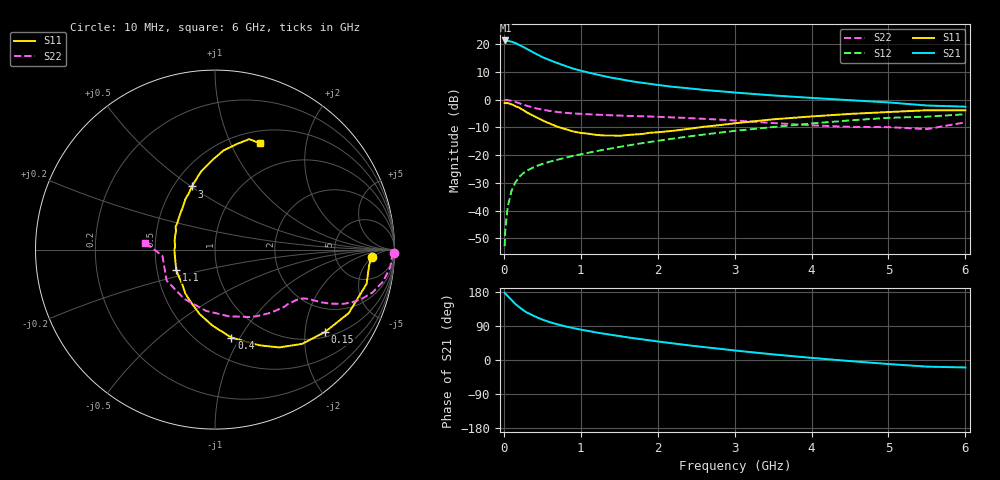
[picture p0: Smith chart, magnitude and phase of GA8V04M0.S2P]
! Infineon Technologies  Discrete & RF Semiconductors
! BF775
! Si NPN RF Bipolar Junction Transistor in SOT23
! VCE = 8 V  IC = 4 mA
! Common Emitter S-Parameters:  May  1996
# GHz  S  MA  R  50
!  f  S11  S21  S12  S22
! GHz  MAG  ANG  MAG  ANG  MAG  ANG  MAG  ANG
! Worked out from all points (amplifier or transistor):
!   36 points, 10 MHz to 6 GHz, reference 50 ohm
!   highest |S21| = 21.3 dB at 20 MHz (marker M1)
!   |S21| within 3 dB of that: start of sweep to 297.3 MHz
!   unconditionally stable (mu >= 1): 922 MHz to 3.067 GHz
!   at 250 MHz: K = 0.42, MSG = 22.8 dB, |S12| = -26.5 dB
!   at 1.4 GHz: K = 1.10, MAG = 10.8 dB, |S12| = -17.5 dB
!   at 6 GHz: K = 0.91, MSG = 1.4 dB, |S12| = -5.3 dB
!   S11 on the Smith chart (normalised r, x): 10 MHz: 13, -5; 150 MHz: 1.15, -2.54; 400 MHz: 0.71, -0.92; 1.1 GHz: 0.63, -0.15; 3 GHz: 0.61, +0.50; 6 GHz: 0.64, +1.30
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0.01  0.8754 -2.6  11.6 177.6  0.0023 90.3  0.9961 -1.1
0.02  0.8634 -5.4  11.63 175.1  0.0047 88.3  0.9869 -2.3
0.05  0.8661 -12.7  11.47 168.8  0.0117 83.5  0.9815 -5.7
0.1  0.8249 -25.4  11.05 158.5  0.0229 77.1  0.9529 -10.8
0.15  0.7654 -36.9  10.45 147.7  0.0325 70.5  0.9086 -15.3
0.2  0.7151 -47.3  9.645 139.6  0.0405 66.2  0.8634 -18.5
0.25  0.6513 -56.8  8.908 131.7  0.0472 62.5  0.8168 -21.1
0.3  0.5878 -65.1  8.194 125.1  0.0528 60.6  0.7741 -23.0
0.4  0.4985 -79.4  6.881 115.4  0.0619 57.2  0.7067 -25.2
0.5  0.4248 -91.7  5.836 106.6  0.0696 55.8  0.6594 -26.4
0.6  0.3693 -103.4  5.129 99.7  0.0765 55.4  0.6243 -27.1
0.7  0.3245 -114.0  4.534 93.9  0.0831 55.7  0.5982 -27.6
0.9  0.2674 -132.4  3.629 84.4  0.0973 56.2  0.5646 -28.8
1.1  0.2437 -152.4  3.072 76.6  0.1109 56.9  0.5451 -30.6
1.3  0.2265 -169.7  2.653 69.5  0.1255 57.2  0.529 -32.4
1.6  0.2304 167.5  2.214 60.0  0.1485 57.4  0.5101 -36.0
2.2  0.275 135.6  1.701 43.8  0.1989 55.6  0.4778 -45.6
3  0.3746 110.2  1.344 25.2  0.2734 50.0  0.4211 -63.1
3.5  0.4421 100.1  1.19 14.8  0.3213 45.1  0.3794 -78.3
4.5  0.5533 85.2  0.977 -2.8  0.4234 33.3  0.3234 -122.1
5.5  0.6438 72.8  0.784 -17.5  0.4937 17.7  0.2948 -173.0
6  0.6435 67.2  0.747 -19.7  0.5457 13.4  0.3901 174.2
